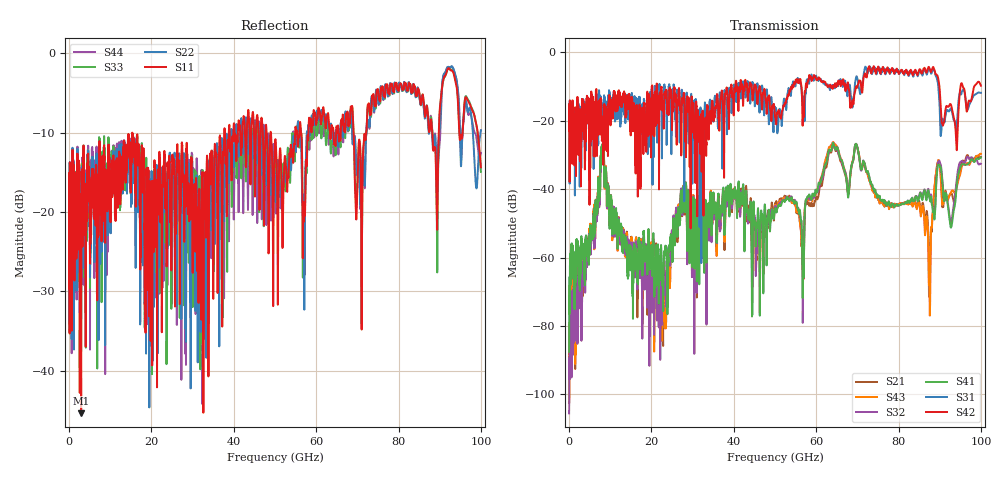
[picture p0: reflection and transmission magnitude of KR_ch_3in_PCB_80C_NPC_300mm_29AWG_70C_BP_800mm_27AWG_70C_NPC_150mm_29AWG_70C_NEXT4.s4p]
# Hz S RI R 45
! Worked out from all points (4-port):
!   4000 points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, 25 MHz to 100 GHz, reference 45 ohm
!   strongest paths, dB at 25 MHz, 25.02 GHz, 50.02 GHz, 75.03 GHz, 100 GHz:
!     S42: -20.7, -20.7, -18.8, -4.2, -9.7
!     S31: -20.6, -12.0, -16.1, -5.0, -11.8
!     S41: -87.5, -61.1, -45.6, -41.8, -30.7
!     S32: -105.5, -52.8, -45.1, -41.8, -32.5
!     S43: -101.7, -55.2, -44.7, -42.8, -29.6
!     S21: -102.5, -56.3, -44.3, -42.9, -30.6
!   lowest |S11| = -45.4 dB at 2.95 GHz (marker M1), VSWR 1.01, Z = 44.7 + j0.377 ohm
!   |S11| at or under -10 dB: start of sweep to 15.35 GHz; 15.35 GHz to 37.69 GHz (22.34 GHz wide, 84.2 % of centre); 49.02 GHz to 54.9 GHz (5.884 GHz wide, 11.3 % of centre)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
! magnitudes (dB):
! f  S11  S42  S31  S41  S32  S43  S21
! 25 MHz  -16.4  -20.7  -20.6  -87.5  -105.5  -101.7  -102.5
! 2.95 GHz  -45.4  -16.5  -19.3  -60.9  -69.9  -72.6  -77.4
! 8.1 GHz  -12.9  -19.0  -18.4  -29.1  -29.8  -29.4  -29.7
! 23 GHz  -14.3  -22.3  -10.8  -62.0  -62.5  -65.0  -64.7
! 27.52 GHz  -12.2  -13.3  -12.3  -46.6  -47.6  -46.4  -47.4
! 87.58 GHz  -9.6  -4.8  -5.0  -42.8  -42.4  -74.7  -63.1
! 100 GHz  -14.3  -9.7  -11.8  -30.7  -32.5  -29.6  -30.6
